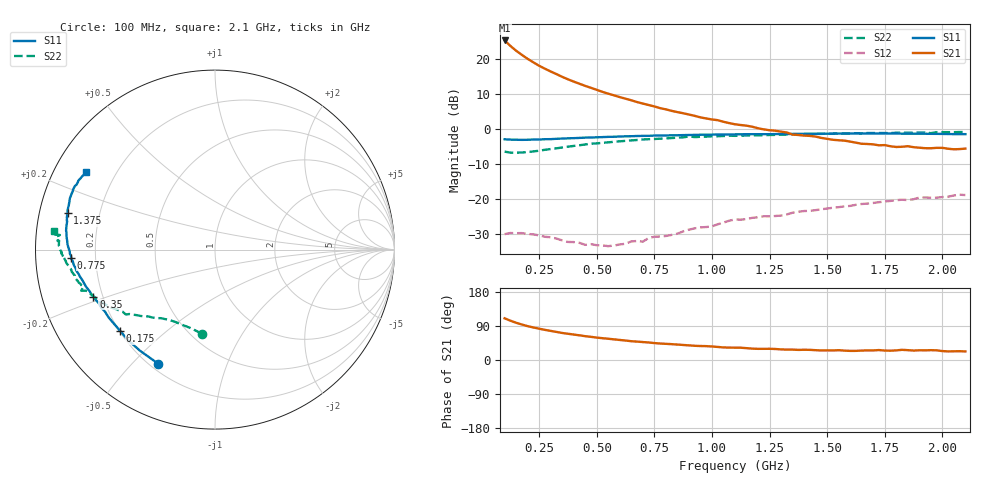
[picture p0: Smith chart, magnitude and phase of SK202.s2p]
!  POLYFET RF DEVICES
!  S PARAMETERS FOR
!  SK202 (Each Side)
!  VDS=28, IDQ=400MA
! S2A2Die, AP pkg,
! Date: Thu Sep 24 14:52:01 1998
# MHZ  S  MA  R  50.0000
! SCATTERING PARAMETERS :
! Freq=MHz Mag[s11] Ang[s11] Mag[s21] Ang[s21] Mag[s12] Ang[s12] Mag[s22] Ang[s22]
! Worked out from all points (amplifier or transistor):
!   81 points, 100 MHz to 2.1 GHz, reference 50 ohm
!   highest |S21| = 25.2 dB at 100 MHz (marker M1)
!   |S21| within 3 dB of that: start of sweep to 151.5 MHz
!   unconditionally stable (mu >= 1): 385.4 MHz to end of sweep
!   at 425 MHz: K = 1.11, MAG = 20.6 dB, |S12| = -32.5 dB
!   at 1.1 GHz: K = 1.24, MAG = 10.6 dB, |S12| = -25.8 dB
!   at 2.1 GHz: K = 1.10, MAG = 4.7 dB, |S12| = -18.9 dB
!   S11 on the Smith chart (normalised r, x): 100 MHz: 0.23, -0.59; 175 MHz: 0.20, -0.36; 350 MHz: 0.16, -0.18; 775 MHz: 0.11, -0.03; 1.375 GHz: 0.08, +0.12; 2.1 GHz: 0.09, +0.27
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100  0.71 -116.6  18.16 110.0  0.03156 22.4  0.4734 -99.0
125  0.7015 -126.6  15.2 103.7  0.03274 17.8  0.4576 -107.8
150  0.6992 -133.9  12.97 98.3  0.03258 15.5  0.4574 -113.9
175  0.6957 -139.4  11.31 93.6  0.03263 13.0  0.4596 -118.7
200  0.6984 -143.9  9.931 89.3  0.03176 11.1  0.4664 -122.6
225  0.7029 -147.5  8.851 85.8  0.03128 11.5  0.4761 -125.5
250  0.7038 -150.6  7.912 82.5  0.03029 11.7  0.4877 -128.4
275  0.711 -152.8  7.188 79.6  0.02891 11.1  0.5025 -130.5
300  0.7128 -155.1  6.562 76.8  0.02851 10.7  0.5152 -132.8
350  0.7262 -158.9  5.501 71.3  0.0257 11.8  0.5419 -136.5
400  0.7362 -161.6  4.709 67.2  0.02432 16.4  0.5702 -140.2
450  0.7487 -164.1  4.09 62.8  0.02219 22.5  0.5983 -143.1
525  0.762 -167.8  3.359 57.5  0.02179 35.9  0.6317 -147.4
600  0.777 -170.6  2.829 52.8  0.0225 48.6  0.6635 -151.0
675  0.7902 -173.5  2.406 48.5  0.02522 58.7  0.693 -154.6
775  0.802 -176.8  1.971 43.5  0.02919 68.4  0.723 -158.6
950  0.8231 177.7  1.456 36.9  0.03936 80.6  0.7698 -165.0
1100  0.8336 173.4  1.16 32.6  0.05109 84.7  0.7939 -169.4
1375  0.8464 166.1  0.8169 26.6  0.06583 87.5  0.8339 -175.6
1450  0.8501 164.6  0.7754 25.9  0.06936 89.4  0.8447 -177.1
1775  0.8578 156.0  0.5638 24.6  0.09372 88.1  0.8693 176.8
2100  0.8393 149.2  0.5222 22.6  0.1137 82.6  0.9008 173.3
